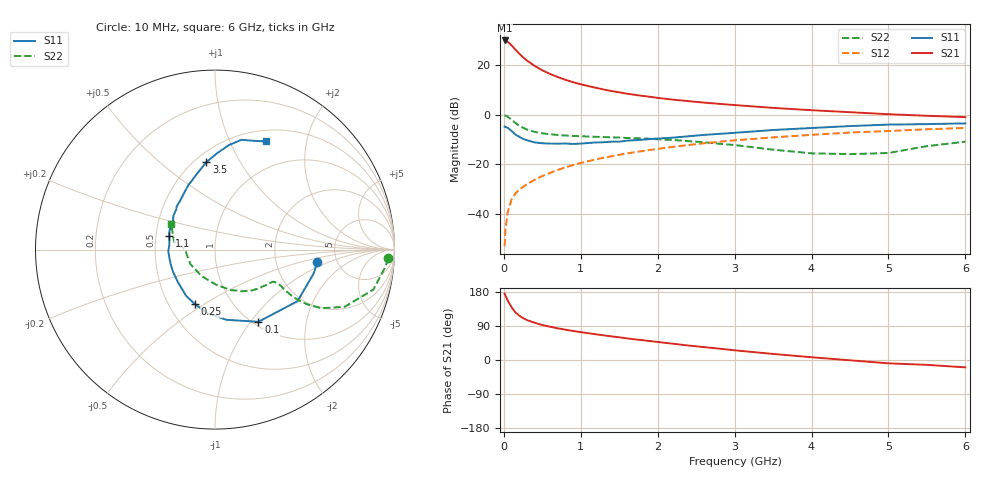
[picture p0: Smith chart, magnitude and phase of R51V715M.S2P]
! SIEMENS Small Signal Semiconductors
! BFR183
! Si NPN RF Bipolar Junction Transistor in SOT23
! VCE = 1.75 V  IC = 15 mA
! Common Emitter S-Parameters:  May  1996
# GHz  S  MA  R  50
!  f  S11  S21  S12  S22
! GHz  MAG  ANG  MAG  ANG  MAG  ANG  MAG  ANG
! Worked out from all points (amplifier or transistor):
!   36 points, 10 MHz to 6 GHz, reference 50 ohm
!   highest |S21| = 30.0 dB at 10 MHz (marker M1)
!   |S21| within 3 dB of that: start of sweep to 129.6 MHz
!   unconditionally stable (mu >= 1): 586 MHz to 2.441 GHz
!   at 250 MHz: K = 0.76, MSG = 26.2 dB, |S12| = -29.2 dB
!   at 1.4 GHz: K = 1.05, MAG = 11.7 dB, |S12| = -16.8 dB
!   at 6 GHz: K = 0.91, MSG = 2.2 dB, |S12| = -5.4 dB
!   S11 on the Smith chart (normalised r, x): 10 MHz: 3.53, -0.74; 100 MHz: 1.06, -1.09; 250 MHz: 0.67, -0.46; 1.1 GHz: 0.59, +0.10; 3.5 GHz: 0.57, +0.73; 6 GHz: 0.63, +1.37
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0.01  0.5745 -7.0  31.53 175.2  0.0022 82.6  0.9672 -2.9
0.02  0.5659 -13.5  31.38 170.3  0.0045 80.3  0.9527 -6.0
0.05  0.5423 -32.0  29.76 157.1  0.0107 76.7  0.91 -14.2
0.1  0.4694 -59.0  25.1 139.3  0.0193 69.3  0.7895 -23.8
0.15  0.3963 -80.7  20.59 125.8  0.0255 66.1  0.6782 -28.8
0.2  0.3578 -96.2  17.12 117.1  0.0306 64.8  0.5989 -30.7
0.25  0.3241 -110.2  14.41 110.5  0.0347 64.4  0.542 -31.2
0.3  0.3044 -121.7  12.4 105.4  0.0393 65.3  0.5007 -31.1
0.4  0.2745 -139.3  9.685 98.3  0.0483 66.7  0.4489 -30.0
0.5  0.2644 -152.2  7.856 92.4  0.0575 67.8  0.4189 -28.9
0.6  0.26 -161.8  6.644 87.8  0.0665 68.4  0.4012 -28.4
0.7  0.2586 -171.3  5.756 83.6  0.0765 68.9  0.389 -28.4
0.8  0.2604 -178.4  5.06 80.0  0.0858 68.5  0.3784 -28.5
0.9  0.2557 174.8  4.526 76.6  0.096 68.3  0.3711 -28.8
1.1  0.2674 163.1  3.767 70.7  0.115 67.5  0.3616 -30.7
1.3  0.2767 153.2  3.217 65.0  0.1352 66.1  0.3519 -32.7
1.6  0.2982 141.1  2.65 57.0  0.1644 63.5  0.3375 -37.1
2.2  0.3429 122.8  2.007 42.9  0.2236 57.5  0.307 -47.8
3.5  0.4892 95.7  1.368 16.0  0.3469 41.1  0.1957 -88.2
4.5  0.5875 82.4  1.12 -0.8  0.435 28.3  0.1593 -149.9
5.5  0.6438 70.3  0.947 -12.8  0.5063 16.3  0.231 169.5
6  0.6652 64.9  0.891 -19.4  0.5388 8.7  0.2839 149.5
